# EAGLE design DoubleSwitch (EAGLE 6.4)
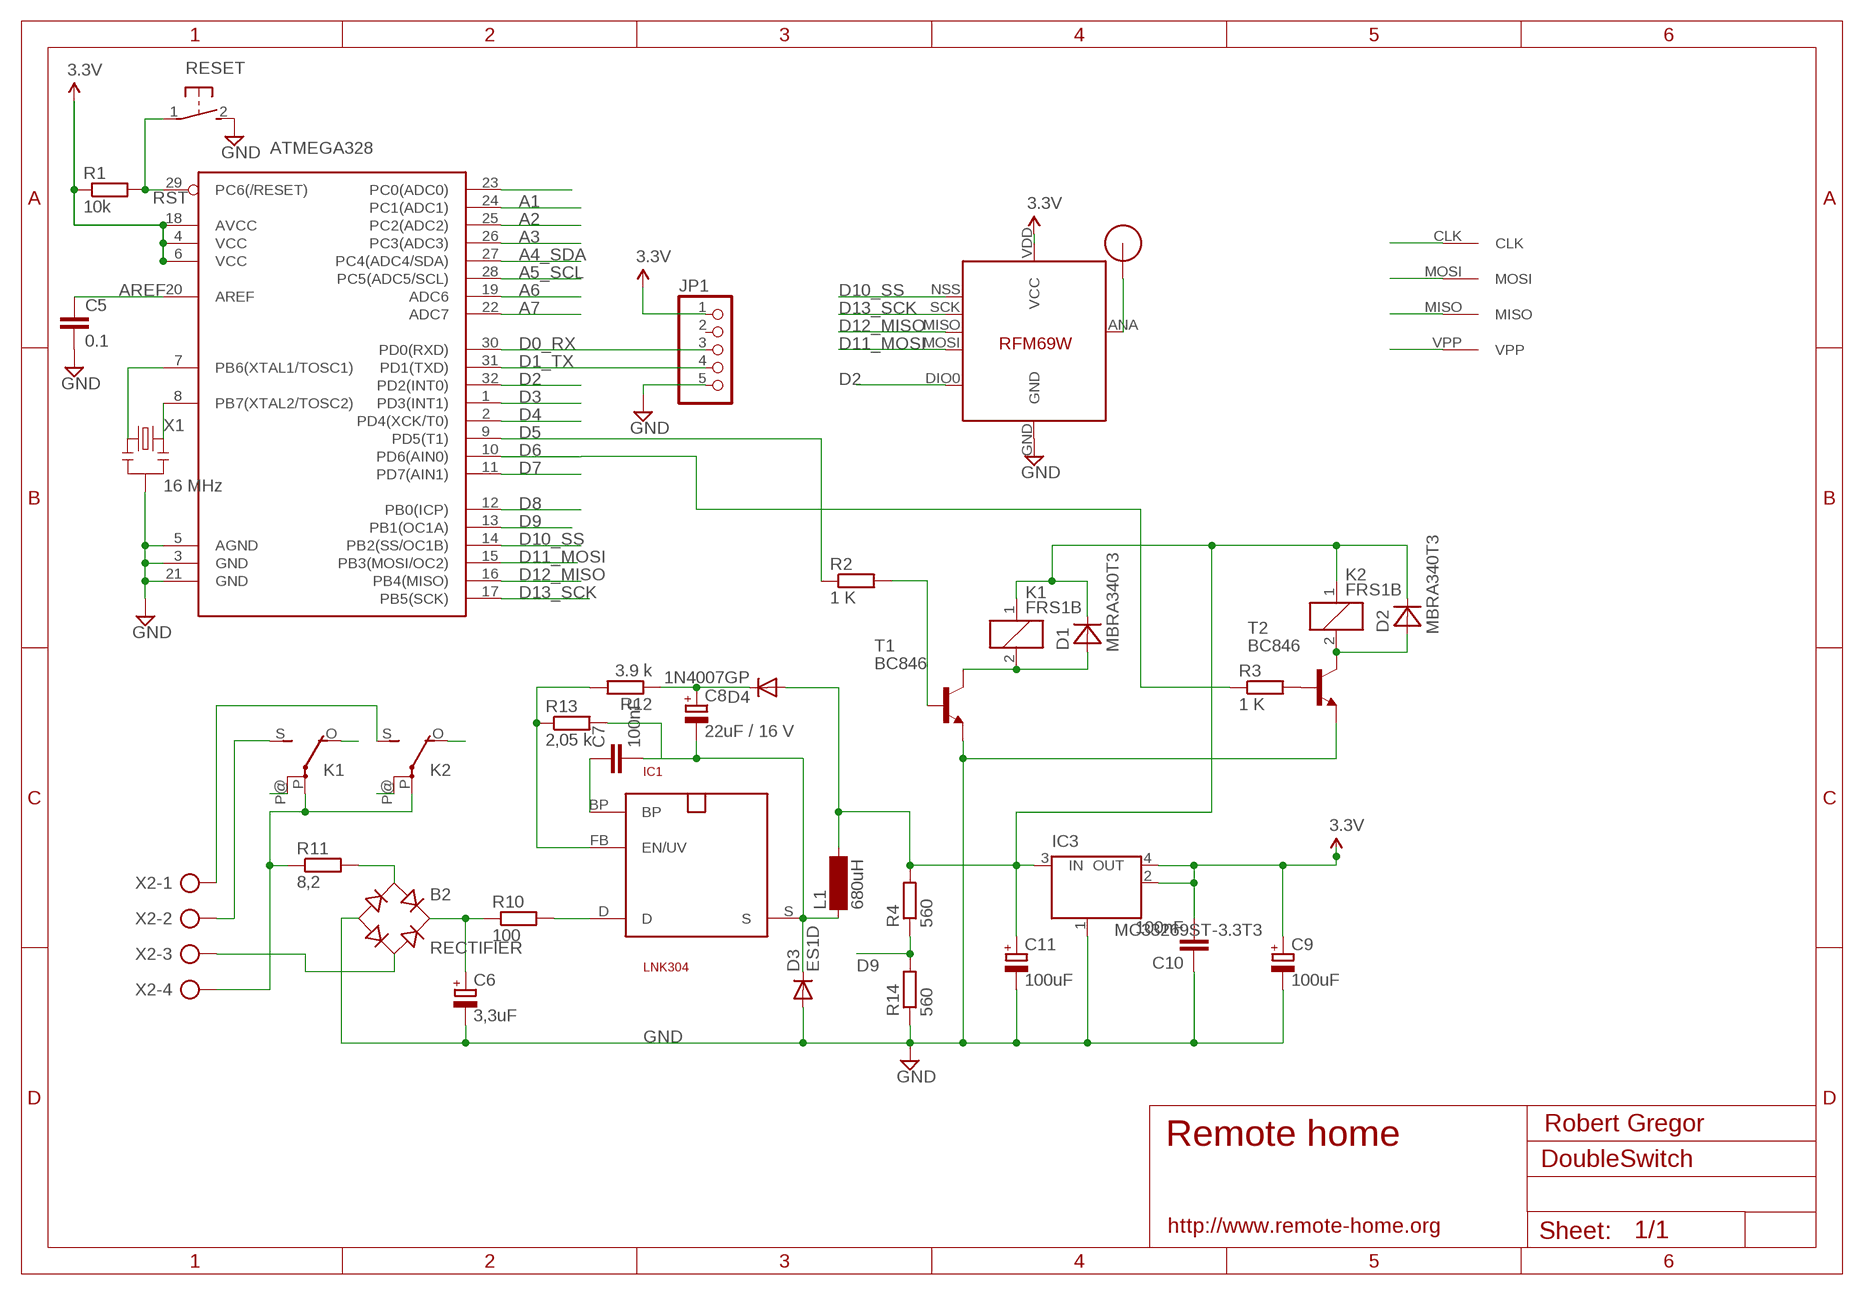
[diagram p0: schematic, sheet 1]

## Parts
ATMEGA328  ATMega-328  ATMEGA168/328TQFP32  [TQFP32-08]
B2  RECTIFIER  RECTIFIER-S40  [TO-269AA]
C5  0.1  C-EUC2012  [C2012]
C6  3,3uF  CPOL-EUE5-10.5  [E5-10,5]
C7  100nF  C-EUC2012  [C2012]
C8  22uF / 16 V  CPOL-EUSMCC  [SMC_C]
C9  100uF  CPOL-EUSMCB  [SMC_B]
C10  100nF  C-EUC2012  [C2012]
C11  100uF  CPOL-EUSMCB  [SMC_B]
D1  MBRA340T3  [SMA]
D2  MBRA340T3  [SMA]
D3  ES1D  DIODE-DO214AC  [DO214AC]
D4  1N4007GP  DIODE-DO214AA  [DO214AA]
IC1  LNK304  SO-8C  [SO-8C]
IC3  MC33269ST-3.3T3  [SOT223]
JP1  PINHD-1X05_2.54-S  [1X05-S]
K1  FRS1B  [FRS1B]
K2  FRS1B  [FRS1B]
L1  680uH  BS11  [BS11]
R1  10k  R-EU_M2012  [M2012]
R2  1 K  R-EU_M2012  [M2012]
R3  1 K  R-EU_M2012  [M2012]
R4  560  R-EU_M2012  [M2012]
R10  100  R-EU_R2512W  [R2512W]
R11  8,2  R-EU_0411/12  [0411/12]
R12  3.9 k  R-EU_M2012  [M2012]
R13  2,05 k  R-EU_M2012  [M2012]
R14  560  R-EU_M2012  [M2012]
RESET  DTSM-3  [DTSM-3]
T1  BC846  [SOT23]
T2  BC846  [SOT23]
U$1  RFM12B_ANTENNA  [RFM12B-ANTENNA]
U$2  AVRHEADERDIP  [AVRHEADER]
U$5  RFM69  [RFM69W-MINPADS]
X1  16 MHz  RESONATORSMD  [RESONATOR-SMD]
X2  AK500/4  [AK500/4]

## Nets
5V: C11.+ D1.C D2.C D4.A IC3.3(IN) K1.1 K2.1 L1.2 R4.2
A0: ATMEGA328.23(PC0(ADC0))
A1: ATMEGA328.24(PC1(ADC1))
A2: ATMEGA328.25(PC2(ADC2))
A3: ATMEGA328.26(PC3(ADC3))
A4_SDA: ATMEGA328.27(PC4(ADC4/SDA))
A5_SCL: ATMEGA328.28(PC5(ADC5/SCL))
A6: ATMEGA328.19(ADC6)
A7: ATMEGA328.22(ADC7)
AREF: ATMEGA328.20(AREF) C5.1
D0_RX: ATMEGA328.30(PD0(RXD)) JP1.3
D1_TX: ATMEGA328.31(PD1(TXD)) JP1.4
D2: ATMEGA328.32(PD2(INT0)) U$5.DIO0
D3: ATMEGA328.1(PD3(INT1))
D4: ATMEGA328.2(PD4(XCK/T0))
D5: ATMEGA328.9(PD5(T1)) R2.1
D6: ATMEGA328.10(PD6(AIN0)) R3.1
D7: ATMEGA328.11(PD7(AIN1))
D8: ATMEGA328.12(PB0(ICP))
D9: ATMEGA328.13(PB1(OC1A)) R4.1 R14.2
D10_SS: ATMEGA328.14(PB2(SS/OC1B)) U$5.NSS(SEL)
D11_MOSI: ATMEGA328.15(PB3(MOSI/OC2)) U$2.MOSI U$5.MOSI
D12_MISO: ATMEGA328.16(PB4(MISO)) U$2.MISO U$5.MISO
D13_SCK: ATMEGA328.17(PB5(SCK)) U$2.CLK U$5.SCK
GND [power]: ATMEGA328.3(GND) ATMEGA328.5(AGND) ATMEGA328.21(GND) B2.- C5.2 C6.- C9.- C10.1 C11.- D3.A IC3.1(GND/ADJ) JP1.5 R14.1 RESET.2 T1.2(E) T2.2(E) U$5.GND X1.2
N678: IC1.FB(EN/UV) R12.2 R13.1
N$1: ATMEGA328.7(PB6(XTAL1/TOSC1)) X1.1
N$2: R2.2 T1.1(B)
N$3: U$1.P$1 U$5.ANA(ANT)
N$4: D2.A K2.2 T2.3(C)
N$5: D1.A K1.2 T1.3(C)
N$6: R3.2 T2.1(B)
N$7 [220V]: K1.S(2:S) X2.2
N$8 [220V]: K1.P(2:P) K2.P(2:P) R11.1 X2.4
N$9 [220V]: B2.AC2 X2.3
N$10: C7.2 C8.- D3.C IC1.S L1.1 R13.2
N$11 [220V]: K1.P@(2:P)
N$12 [220V]: K2.S(2:S) X2.1
N$13 [220V]: IC1.D R10.2
N$14 [220V]: B2.+ C6.+ R10.1
N$15 [220V]: B2.AC1 R11.2
N$16 [220V]: K2.P@(2:P)
N$17 [220V]: K1.O(2:O)
N$18: C7.1 IC1.BP
N$19 [220V]: K2.O(2:O)
N$20: C8.+ D4.C R12.1
N$21: ATMEGA328.8(PB7(XTAL2/TOSC2)) X1.3
RST: ATMEGA328.29(PC6(/RESET)) R1.2 RESET.1 U$2.VPP
VCC: ATMEGA328.4(VCC) ATMEGA328.6(VCC) ATMEGA328.18(AVCC) C9.+ C10.2 IC3.2(OUT) IC3.4(OUT) JP1.1 R1.1 U$5.VDD(VCC) ; supply symbol labelled 3.3V
Unconnected: JP1.2

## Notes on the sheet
- Robert Gregor
- Remote home
- http://www.remote-home.org

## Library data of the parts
ATMEGA328 = LowPowerLab:ATMEGA168/328: Atmel 32-pin 8-bit micro, 16k flash.
B2 = rectifier:RECTIFIER-: Rectifier
C5 C7 C10 = resistor:C-EU: CAPACITOR, European symbol
C6 C8 C9 C11 = resistor:CPOL-EU: POLARIZED CAPACITOR, European symbol
D1 D2 = diode:MBRA340T3: Surface Mount Schottky Power Rectifier
D3 D4 = diode:DIODE-: DIODE
IC1 = powerint:SO-8C: 700V MOSFET für Schaltnetz-Trafos. Pin 3 fehlt. SMD
IC3 = linear:MC33269ST*: Adjustable Output Low Dropout Voltage Regulator 800 mA Source: http://www.onsemi.com/pub/Collateral/MC33269-D.PDF
JP1 = pinhead-2:PINHD-1X05: PIN HEADER
K1 K2 = relay:FRS1B: RELAY 1 x switch, same as V23101-D6-A201, Siemens; OC_FARNELL: unknown; OC_NEWARK: unknown
L1 = inductor-neosid:BS: INDUCTOR; OC_FARNELL: unknown; OC_NEWARK: unknown
R1-R4 R10-R14 = resistor:R-EU_: RESISTOR, European symbol
RESET = switch-tact:DTSM-3
T1 T2 = transistor:BC846: NPN TRANSISTOR
U$1 = LowPowerLab:RFM12B_ANTENNA
U$2 = RemoteHome:AVRHEADER
U$5 = LowPowerLab:RFM69
X1 = SparkFun:RESONATOR: Resonator Small SMD resonator. This is the itty bitty 10/20MHz resonators with built in caps. CSTCE10M0G55 and CSTCE20M0V53. Footprint has been reviewed closely but hasn't been tested yet.
X2 = con-ptr500:AK500/4: CONNECTOR; OC_FARNELL: unknown; OC_NEWARK: unknown

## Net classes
1 power: width 0.381 mm, clearance 0.254 mm
2 220V: width 0.381 mm, clearance 0.508 mm

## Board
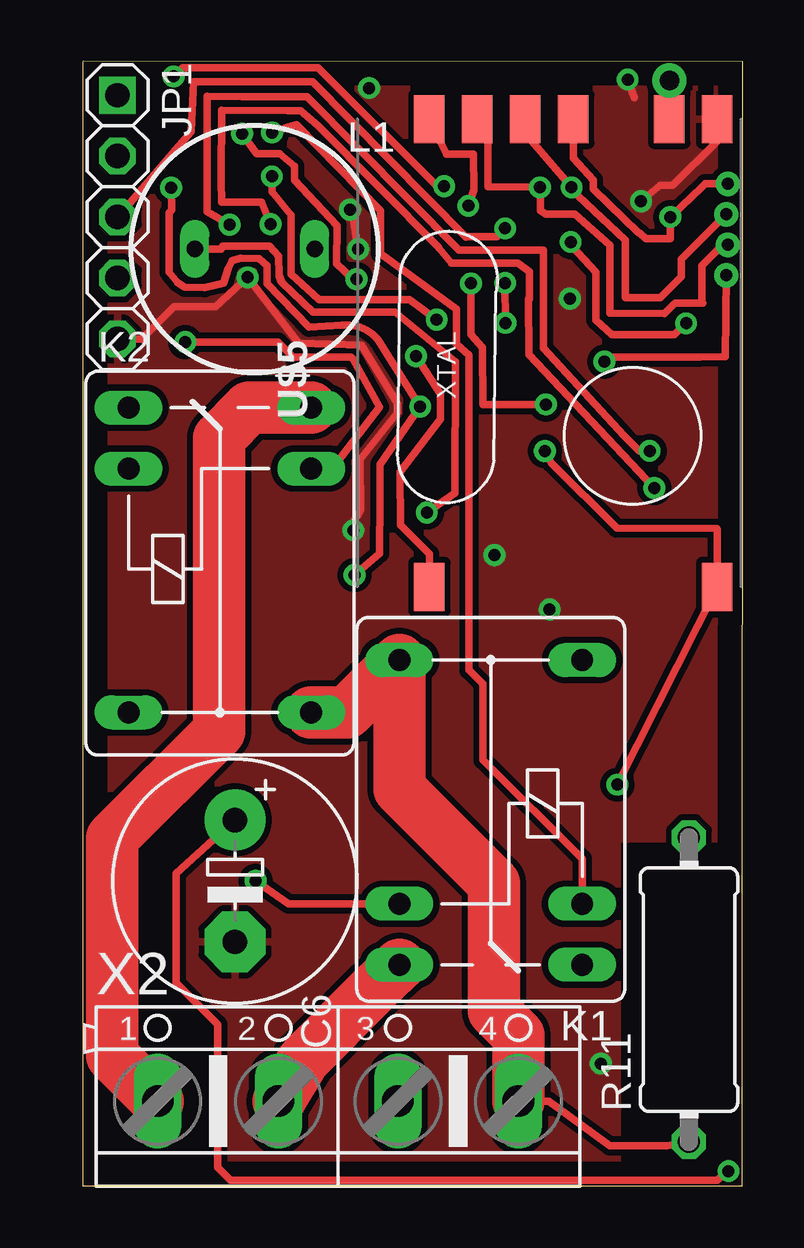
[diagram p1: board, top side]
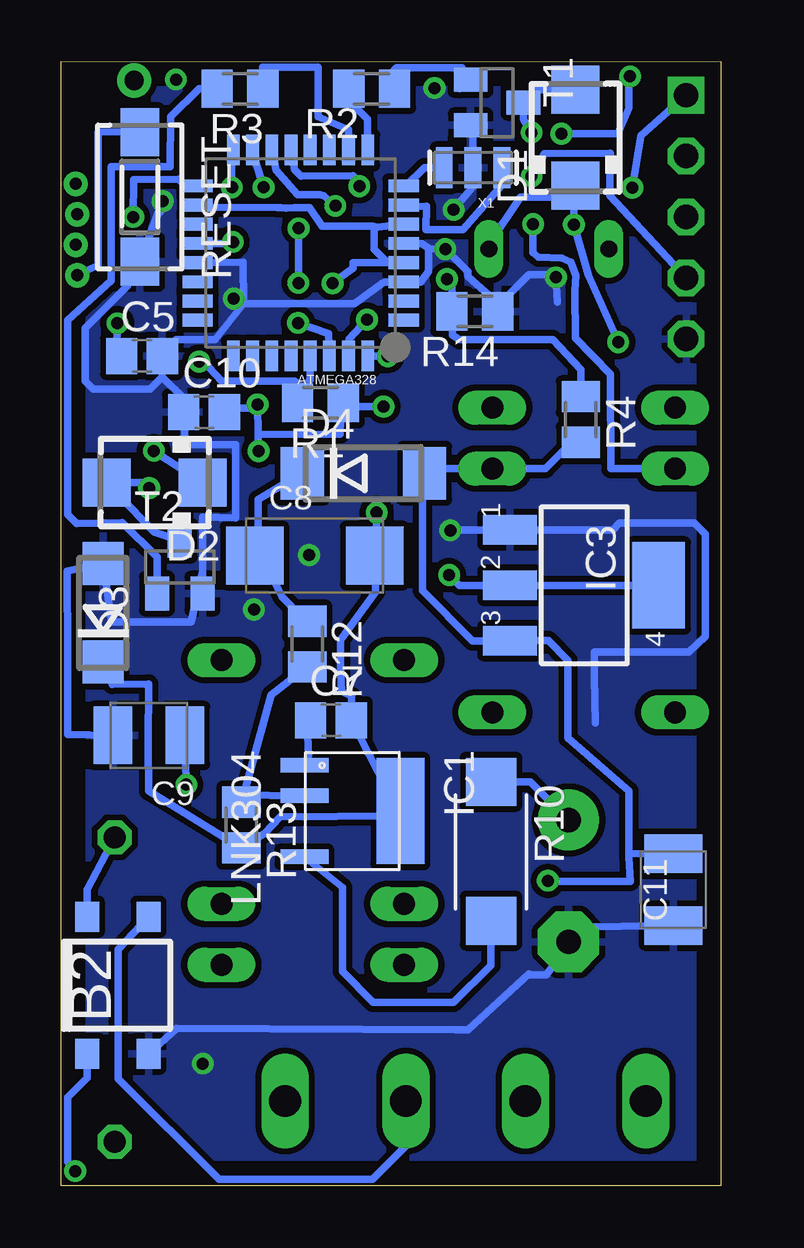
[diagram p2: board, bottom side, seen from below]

Size 27.51 x 46.86 mm. Coordinates in mm from the lower left corner, seen from the top.
Outline: 0.01,46.86 27.51,46.86 27.51,46.78 27.5,0 0,0 0,46.86
Copper layers (1*16): Top 0.035mm / dielectric 1.5mm / Bottom 0.035mm
Design rules "default": minimum track width 10mil, minimum drill 24mil, track to track 8mil, track to pad 8mil, pad to pad 8mil, via to via 8mil, smd to smd 8mil, copper to edge 40mil, drill to drill 8mil, minimum pad ring 10mil, minimum via ring 8mil, stop-mask expansion 4mil, vias tented up to drill 0mil, thermal gap 10mil

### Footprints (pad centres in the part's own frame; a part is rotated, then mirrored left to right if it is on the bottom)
TQFP32-08 = smd 1.27 x 0.533: 1 -4.293,2.8; 2 -4.293,2; 3 -4.293,1.2; 4 -4.293,0.4; 5 -4.293,-0.4; 6 -4.293,-1.2; 7 -4.293,-2; 8 -4.293,-2.8; 17 4.293,-2.8; 18 4.293,-2; 19 4.293,-1.2; 20 4.293,-0.4; 21 4.293,0.4; 22 4.293,1.2; 23 4.293,2; 24 4.293,2.8 | smd 0.533 x 1.27: 9 -2.8,-4.293; 10 -2,-4.293; 11 -1.2,-4.293; 12 -0.4,-4.293; 13 0.4,-4.293; 14 1.2,-4.293; 15 2,-4.293; 16 2.8,-4.293; 25 2.8,4.293; 26 2,4.293; 27 1.2,4.293; 28 0.4,4.293; 29 -0.4,4.293; 30 -1.2,4.293; 31 -2,4.293; 32 -2.8,4.293
TO-269AA = smd 1 x 1.25: + -1.28,-2.855; - 1.28,-2.855; AC1 -1.28,2.855; AC2 1.28,2.855
C2012 = smd 1.3 x 1.5: 1 -0.85,0; 2 0.85,0
E5-10,5 = drill 1.016 pad 2.54: + -2.54,0 | drill 1.016 pad 2.54 octagon: - 2.54,0
SMC_C = smd 2.4 x 2.4: + -2.5,0; - 2.5,0
SMC_B = smd 1.6 x 2.4: + -1.5,0; - 1.5,0
SMA = smd 2 x 2: A 2,0; C -2,0
DO214AC = smd 1.8 x 1.7: A 2.05,0; C -2.05,0
DO214AA = smd 1.8 x 2.2: A 2.55,0; C -2.55,0
SO-8C = smd 0.6 x 2: BP -1.905,-2; D 1.905,-2; FB -0.635,-2 | smd 4.41 x 2: S 0,2
SOT223 = smd 1.219 x 2.235: 1 -2.311,-3.099; 2 0,-3.099; 3 2.311,-3.099 | smd 3.6 x 2.2: 4 0,3.099
1X05-S = drill 1.016 square: 1 -5.08,0 | drill 1.016 octagon: 2 -2.54,0; 3 0,0; 4 2.54,0; 5 5.08,0
FRS1B = drill 0.914 long: 1 0,3.81; 2 0,-3.81; O -2.54,-3.81; P 10.16,3.81; P@ 10.16,-3.81; S -2.54,3.81
BS11 = drill 0.7 long: 1 -2.5,0; 2 2.5,0
M2012 = smd 1.3 x 1.6: 1 -0.95,0; 2 0.95,0
R2512W = smd 2 x 2.1: 1 -2.896,0; 2 2.896,0
0411/12 = drill 0.914 octagon: 1 -6.35,0; 2 6.35,0
DTSM-3 = smd 2 x 1.6: 1 -2.7,0; 2 2.7,0
SOT23 = smd 1 x 1.4: 1 -0.95,-1.1; 2 0.95,-1.1; 3 0,1.1
RFM12B-ANTENNA = drill 0.8 pad 1.422: P$1 0,0
AVRHEADER = drill 0.5: CLK 2.54,0; MISO 1.27,0.07; MOSI 0,0; VPP -1.27,0.072
RFM69W-MINPADS = smd 2 x 1.27: ANA 8,-5; DIO0 -11.5,5; GND 8,-7; MISO 8,1; MOSI 8,3; NSS 8,5; SCK 8,-1; VDD -11.5,-7
RESONATOR-SMD = smd 0.7 x 1.7: 1 -1.2,0; 2 0,0; 3 1.2,0
AK500/4 = drill 1.321 long: 1 -7.518,0; 2 -2.489,0; 3 2.489,0; 4 7.518,0

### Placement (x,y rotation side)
ATMEGA328  17.52,38.88 180 bottom
B2  25.14,8.36 0 bottom
C5  24.13,34.59 0 bottom
C6  6.34,12.7 270 top
C7  16.25,19.4 0 bottom
C8  16.93,26.27 0 bottom
C9  23.84,18.77 180 bottom
C10  21.54,32.24 0 bottom
C11  1.97,12.34 270 bottom
D1  6.06,43.68 90 bottom
D2  23.6,29.31 180 bottom
D3  25.74,23.88 90 bottom
D4  14.9,29.7 0 bottom
IC1  15.35,15.62 270 bottom
IC3  5.69,25.03 270 bottom
JP1  1.44,40.38 270 top
K1  17.01,11.75 90 top
K2  5.71,29.89 270 top
L1  7.17,39.05 0 top
R1  16.69,32.63 180 bottom
R2  14.55,45.73 0 bottom
R3  20.04,45.73 180 bottom
R4  5.83,31.94 270 bottom
R10  9.58,13.94 270 bottom
R11  25.27,8.18 90 top
R12  17.24,22.58 270 bottom
R13  19.98,15.03 270 bottom
R14  10.25,36.44 180 bottom
RESET  24.22,41.21 270 bottom
T1  9.33,45.15 270 bottom
T2  22.55,25.79 0 bottom
U$1  24.46,46.07 0 top
U$2  26.9,39.22 90 top
U$5  19.45,36.46 90 top
X1  10.33,42.44 180 bottom
X2  10.64,3.53 0 top

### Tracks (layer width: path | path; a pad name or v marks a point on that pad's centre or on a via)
5V  (via drill 0.5)
  Top 0.305: K1.1 8.57,11.75 v7.21,12.71 | v6.12,40.06 5.18,40.61 5.17,45.41 6.65,45.4 9.34,45.39 15.69,39.01 19.2,39.01 19.21,34.92 22.59,31.25 23.2,30.63 v23.63,30.63 | v4.27,35.16 8.14,35.16 8.76,34.55 11.17,34.55 11.26,34.46 12.37,32.45 10.36,29.86 K2.1
  Bottom 0.305: 3.82,13.86 3.82,13.69 3.77,12.68 7.13,12.68 7.19,12.7 v7.21,12.71 | 3.82,13.86 3.82,16.47 6.37,18.67 6.37,21.9 7.19,22.73 IC3.3 10.34,22.72 12.43,24.8 12.43,29.61 D4.A 12.15,29.89 K2.1 7.3,29.89 6.21,30.99 R4.2 | 6.12,40.87 v6.12,40.06 5.52,37.95 v4.27,35.17 v4.27,35.16 | 6.12,40.87 D1.C | 6.12,40.87 6.13,41.21 8.35,41.21 9.67,39.25 L1.2 | D2.C v23.63,30.63 | C11.+ 3.82,13.86
AREF  (via drill 0.5)
  Top 0.305: v20.34,39.34 20.39,39.17 21.38,38.09 21.38,36.07 22.06,35.48 24.66,35.48 v25.15,35.95
  Bottom 0.305: ATMEGA328.20 20.64,39.28 v20.34,39.34 | v25.15,35.95 25.18,34.79 C5.1
D0_RX  (via drill 0.5)
  Top 0.305: v17.61,37.63 v17.62,35.97 | JP1.3 4.52,43.93 4.61,46.01 9.57,46.01 15.98,39.54 16,39.55 17.27,39.55 17.61,39.89 v17.61,39.91
  Bottom 0.305: v17.61,39.91 v17.61,37.63 | v17.62,35.97 16.34,35.52 ATMEGA328.30
D1_TX  (via drill 0.5)
  Top 0.305: v7.88,42.07 7.88,41.43 8.69,40.47 8.69,38 9.85,36.95 13.62,36.94 v14.75,36.1
  Bottom 0.305: v7.88,42.07 7.34,43.01 4.61,43.03 4.62,41.28 JP1.4 | v14.75,36.1 15.24,35.56 15.51,35.29 15.51,34.6 ATMEGA328.31
D2  (via drill 0.5)
  Top 0.305: U$5.DIO0 14.45,26.34 13.24,27.54 13.21,29.75 14.92,31.95 14.92,33 v13.88,34.58
  Bottom 0.305: v13.88,34.58 14.71,34.58 ATMEGA328.32
D5
  Bottom 0.305: 14.77,43.22 ATMEGA328.9 14.72,44.47 15.5,45.25 R2.1
D6
  Bottom 0.305: ATMEGA328.10 15.52,44.02 16.79,44.56 16.79,46.62 19.1,46.62 19.11,45.78 R3.1
D9  (via drill 0.5)
  Top 0.305: v11.41,37.79 11.24,37.8 10.59,38.43 10.6,40.02 8.82,41.91 8.82,42.49 8.19,43.01 7.25,43.03 v6.64,43.85 | v3.78,46.24 | v3.78,46.24 4.15,46.61 9.8,46.61 14.75,41.68 v15.07,41.66
  Bottom 0.305: R4.1 5.83,34.02 6.99,35.27 10.9,35.27 11.18,35.46 11.18,36.2 R14.2 11.2,37.98 v11.41,37.79 | v6.64,43.85 4.29,43.86 3.84,44.91 3.84,46.18 v3.78,46.24 | ATMEGA328.13 17.77,42.34 17.5,42.07 15.33,42.09 v15.07,41.66
D10_SS  (via drill 0.5)
  Top 0.305: U$5.NSS 15.17,42.99 16.29,42.99 16.31,41.52 v16.07,40.84
  Bottom 0.305: v16.07,40.84 16.55,41.27 16.7,41.31 17.64,41.31 18.54,42.33 18.7,43.16 ATMEGA328.14
D11_MOSI  (via drill 0.5)
  Top 0.305: U$5.MOSI 16.9,43.64 16.9,41.65 v19.05,41.62 19.08,41.61 19.08,40.65 19.31,40.5 20.52,40.5 21.97,39.2 21.97,36.38 24.25,36.36 24.61,36.7 24.7,36.79 25.85,36.79 25.82,36.82 25.82,38.35 26.69,39.22 U$2.MOSI
  Bottom 0.305: v19.05,41.62 19.54,43.15 ATMEGA328.15
D12_MISO  (via drill 0.5)
  Top 0.305: U$5.MISO 18.45,43.85 v20.38,41.62 20.64,41.27 22.61,39.41 22.62,37.02 24.08,37.02 24.96,37.91 24.96,38.62 U$2.MISO
  Bottom 0.305: v20.38,41.62 20.42,43 ATMEGA328.16
D13_SCK  (via drill 0.5)
  Top 0.305: U$5.SCK 20.45,42.83 21.28,41.92 21.28,41.53 23.16,39.74 23.22,39.71 23.47,39.49 24.48,39.49 v24.49,40.38 25.83,41.64 25.95,41.76 U$2.CLK
  Bottom 0.305: ATMEGA328.17 22.34,41.68 22.6,41.95 24.48,41.93 v24.49,40.38
GND  (via drill 0.5)
  Top 0.305: v11.28,27.32 11.28,27.67 11.58,28.17 11.57,30.27 13.12,32.23 13.13,32.6 11.63,35.04 9,35.13 v6.87,37.87 5.53,36.64 3.8,36.64 2.46,35.3 JP1.5 | v11.13,40.69 11.24,40.54 v11.48,39.04 | U$5.GND 26.45,43.55 24.61,41.71 24.08,41.71 v23.27,41.04 | v22.71,46.11 22.99,45.36
  Bottom 0.305: B2.- 22.69,6.55 11.04,6.5 10.55,6.49 8,8.82 7.99,8.79 7.26,8.79 6.34,10.01 C6.- 6.34,10.78 C11.- | 5.23,19.29 5.26,21.18 5.26,22.25 1.33,22.25 0.65,22.9 0.65,27.16 1.1,27.62 4.22,27.62 4.5,27.34 IC3.1 11.26,27.34 v11.28,27.32 | T1.2 10.33,44.26 X1.2 10.33,41.65 v11.13,40.69 | ATMEGA328.21 19.91,38.49 19.9,36.78 | 19.9,36.78 15.26,36.76 14.11,37.62 13.99,37.66 13.24,37.66 ATMEGA328.3 13.21,37.66 12.53,37.66 12.18,38.11 12.18,38.59 12.18,39.05 12.12,39.04 | ATMEGA328.5 12.45,39.28 12.12,39.04 | 6.81,36.84 v6.87,37.87 6.86,37.97 8,37.97 9.3,36.67 R14.1 9.3,36.8 10.53,37.89 10.53,38.1 v11.48,39.04 11.68,39.05 12.12,39.04 | 19.9,36.78 21.07,35.27 22.7,35.27 23.09,34.82 C5.2 23.28,33.7 | 23.28,33.7 22.36,32.78 C10.1 22.36,32.52 22.36,30.9 20.22,30.89 20.22,27.84 21.61,27.87 21.61,27.88 T2.2 21.61,25.61 22.09,23.5 25.4,23.5 D3.A 27.24,25.62 27.24,25.34 27.22,22.43 27.22,18.81 C9.- | 23.28,33.7 23.78,33.2 26.16,33.2 26.5,33.54 26.5,35.75 24.73,37.53 RESET.2 v23.27,41.04 23.34,40.62 23.37,40.59
  other vias: 21.6,5.09 11.93,45.76 17.16,26.29 19.46,24.02 20.3,36.98
  pour Top: 0.17,46.7 27.34,46.7 27.34,14.46 22.28,14.46 22.28,0.15 0.15,0.15 0.15,46.62
  pour Bottom: 0.23,46.7 27.35,46.66 27.35,0.16 0.18,0.16 0.15,46.66
N678
  Bottom 0.305: IC1.FB 18.18,16.25 19.44,16.28 19.69,16.28 R13.1 18.75,20.46 R12.2
N$1
  Bottom 0.305: ATMEGA328.7 13.22,40.84 13.18,40.79 12.27,40.82 12.28,39.85 10.75,39.86 9.12,41.71 X1.1
N$2
  Bottom 0.305: T1.1 10.88,45.73 10.88,46.5 10.79,46.59 13.51,46.59 13.61,46.49 13.61,45.73 R2.2
N$3
  Top 0.305: U$5.ANA 24.45,46.06 U$1.P$1
N$4  (via drill 0.5)
  Top 0.305: v7.82,40.08 7.45,41 5.78,41.01 5.77,41.92 5.78,44.84 8.54,44.82 9.08,44.82 9.8,44.18 14.82,39.12 14.85,39.08 15.38,38.47 18.15,38.47 18.61,38.11 18.61,36.96 18.59,36.96 18.59,34.65 v23.83,29.08
  Bottom 0.305: K2.2 4.58,29.89 4.6,33.84 6.06,35.34 6.08,37.31 6.05,37.94 6.26,38.49 6.62,38.67 7.6,38.7 7.83,38.89 v7.82,40.08 | T2.3 23.61,27.25 D2.A 24.06,29.31 v23.83,29.08
N$5  (via drill 0.5)
  Top 0.305: K1.2 20.82,13.63 16.69,17.76 16.69,20.91 16.1,21.51 16.09,34.63 15.59,35.07 15.58,36.53 12.41,38.86 12.41,40.65 8.9,44.23 8.53,44.13 v7.89,43.9
  Bottom 0.305: v7.89,43.9 8.22,44.45 T1.3 7.73,45.67 D1.A
N$6
  Bottom 0.305: R3.2 21.74,45.73 22.94,44.57 22.95,42.48 25.41,42.48 25.41,37.73 27.23,36.07 27.23,33.54 27.22,33.5 27.22,27.97 26.85,27.61 24.95,27.65 23.5,26.21 T2.1
N$7
  Top 2.184: X2.2 9.2,5.26 12.12,8.18 13.08,9.1 K1.S
N$8
  Top 0.305: X2.4 19.44,3.53 21.98,1.67 24.34,1.67 R11.1
  Top 2.184: X2.4 18.16,6.27 17.13,7.3 17.13,12.6 13.2,16.54 K1.P 11.02,19.73 K2.P
N$9
  Bottom 0.305: X2.3 13.13,1.66 14.52,0.27 20.91,0.27 25.13,4.47 25.13,9.84 B2.AC2
N$10  (via drill 0.5)
  Top 0.305: v14.34,28.06 15.52,28.87 15.54,34.36 13.01,36.41 9.6,36.41 8.29,37.67 8.19,37.94 8.18,37.97 8.16,38.74 7.78,39.16 5.83,39.16 5.76,39.05 L1.1
  Bottom 0.305: v14.34,28.06 14.38,25.86 C8.- 14.39,24.74 15.84,22.76 15.84,21.43 15.81,20.62 15.38,20.39 C7.2 13.56,15.83 IC1.S 13.6,15.41 18.38,15.37 19.03,14.68 R13.2 20,14.07 23.85,16.45 23.87,18.41 23.86,20.91 25.38,20.9 D3.C
N$12
  Top 2.184: K2.S 6.93,32.43 5.68,31.18 5.68,18.95 1.23,14.5 1.23,5.42 X2.1
N$13
  Bottom 0.305: R10.2 9.58,9.19 11.15,7.64 14.49,7.64 15.77,8.93 15.77,12.44 IC1.D
N$14  (via drill 0.5)
  Top 0.305: v26.92,0.61 27.03,0.8 26.46,0.23 6.16,0.23 5.61,0.78 5.61,6.72 3.9,8.46 3.9,13.02 C6.+
  Bottom 0.305: R10.1 7.93,16.83 C6.+ | B2.+ 26.42,4.49 27.22,3.69 27.22,0.99 v26.92,0.61
N$15
  Bottom 0.305: B2.AC1 26.42,11.19 26.41,11.18 26.41,12.36 R11.2
N$18
  Bottom 0.305: C7.1 17.23,18.78 17.18,17.91 17.38,17.56 IC1.BP
N$20
  Bottom 0.305: R12.1 17.44,23.67 18.29,24.55 18.93,25.85 C8.+ 19.39,25.89 19.29,25.99 19.29,28.61 D4.C
N$21
  Bottom 0.305: ATMEGA328.8 13.11,41.68 12.35,42.44 X1.3 | X1.3
RST  (via drill 0.5)
  Top 0.305: U$2.VPP 26.79,34.55 25.73,34.55 22.11,34.55 v21.74,34.35
  Bottom 0.305: ATMEGA328.29 17.12,33.57 17.42,33.27 | 17.42,33.27 17.42,32.51 R1.2 | v21.74,34.35 21.57,34.38 20.81,33.54 17.77,33.54 17.42,33.27 | 24.18,43.28 RESET.1 25.95,43.94 25.96,43.27 25.96,38.37 U$2.VPP
VCC  (via drill 0.5)
  Top 0.305: v11.32,25.45 12.37,26.36 12.38,28.65 12.38,30.06 v14.06,32.48 12.38,35.16 arc61 10.81,35.87 9.44,35.8 7.68,37.6 7.68,38.35 7.35,38.64 6.57,38.67 6.22,38.55 6.05,38.23 5.87,37.62 5.07,37.45 4.25,37.45 3.95,37.64 3.59,38.08 3.59,40.56 3.7,40.67 v3.68,41.6 | v16.18,37.62 16.18,35.48 16.66,34.94 16.68,32.56 v19.31,32.57 | v19.26,30.62 19.54,30.13 22.26,27.41 26.44,27.4 26.45,27.33 U$5.VDD v22.28,16.72
  Bottom 0.305: IC3.4 IC3.2 10.9,25.03 v11.32,25.45 | ATMEGA328.6 14.32,39.96 | 14.32,39.96 14.51,40 15.27,40 16.61,40 17.14,40.77 17.78,40.77 18.12,40.76 18.34,40.78 18.47,40.77 21.79,40.78 ATMEGA328.18 | 14.32,39.96 14.45,39.89 14.45,39.03 13.89,38.48 ATMEGA328.4 15.33,38.48 15.33,38.25 v16.18,37.62 | v14.06,32.48 15.75,32.48 R1.1 15.82,32.47 15.87,31.34 19.3,31.3 | 19.3,31.3 v19.26,30.62 | 19.3,31.3 v19.31,32.57 19.28,32.43 20.49,32.43 20.53,32.46 C10.2 | JP1.1 3.33,43.76 v3.68,41.6 | C9.+ v22.28,16.72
